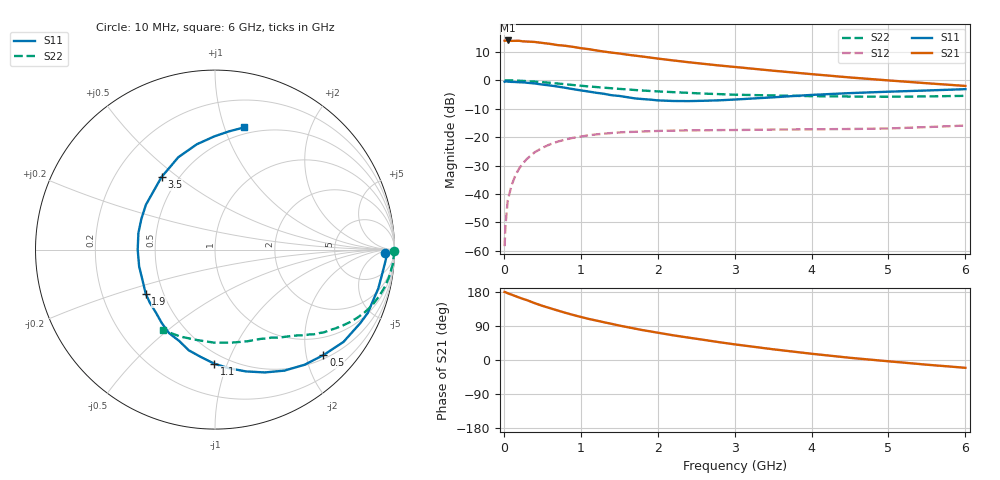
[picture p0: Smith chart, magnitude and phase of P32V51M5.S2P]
! SIEMENS Small Signal Semiconductors
! BFP181
! Si NPN RF Bipolar Junction Transistor in SOT143
! VCE = 2.5 V  IC = 1.5 mA
! Common Emitter S-Parameters:  March  1996
# GHz  S  MA  R  50
!  f  S11  S21  S12  S22
! GHz  MAG  ANG  MAG  ANG  MAG  ANG  MAG  ANG
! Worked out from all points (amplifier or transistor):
!   36 points, 10 MHz to 6 GHz, reference 50 ohm
!   highest |S21| = 14.1 dB at 50 MHz (marker M1)
!   |S21| within 3 dB of that: start of sweep to 1.086 GHz
!   unconditionally stable (mu >= 1): 2.69 GHz to end of sweep
!   at 250 MHz: K = 0.11, MSG = 21.4 dB, |S12| = -29.2 dB
!   at 1.4 GHz: K = 0.58, MSG = 14.2 dB, |S12| = -18.6 dB
!   at 6 GHz: K = 1.18, MAG = 4.4 dB, |S12| = -15.9 dB
!   S11 on the Smith chart (normalised r, x): 10 MHz: 31, -11; 500 MHz: 0.58, -2.34; 1.1 GHz: 0.42, -0.90; 1.9 GHz: 0.40, -0.25; 3.5 GHz: 0.40, +0.44; 6 GHz: 0.44, +1.17
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0.01  0.9447 -1.2  4.986 179.5  0.0012 90.4  0.9978 -0.3
0.02  0.9578 -1.9  5.023 179.0  0.0026 81.4  0.9975 -0.9
0.05  0.9502 -4.4  5.041 176.2  0.0076 89.5  0.9961 -2.0
0.1  0.9394 -9.4  4.957 172.5  0.0141 81.9  0.9955 -4.1
0.2  0.9248 -18.2  4.973 164.8  0.0281 78.6  0.9846 -8.2
0.4  0.8814 -35.7  4.743 150.0  0.054 67.7  0.9507 -15.9
0.5  0.8429 -44.2  4.56 143.0  0.0647 62.3  0.929 -19.5
0.6  0.8129 -52.1  4.389 136.8  0.0747 58.0  0.9046 -22.7
0.8  0.7386 -67.9  4.059 124.6  0.0908 49.8  0.8542 -28.2
0.9  0.7 -75.8  3.886 118.9  0.0972 45.9  0.8278 -30.7
1.1  0.6353 -90.4  3.549 108.6  0.1078 39.7  0.7812 -35.1
1.3  0.5799 -104.6  3.215 99.7  0.115 34.0  0.7429 -38.8
1.5  0.5314 -118.7  2.971 90.9  0.1208 29.8  0.7068 -42.0
1.8  0.4684 -140.8  2.628 79.0  0.1258 24.6  0.6624 -46.2
1.9  0.4582 -147.3  2.524 75.6  0.1267 22.8  0.6496 -47.7
2.2  0.4329 -167.6  2.244 65.2  0.1302 19.0  0.6196 -51.8
2.8  0.4445 157.4  1.826 47.0  0.133 13.8  0.5721 -60.0
3.5  0.5022 126.4  1.479 28.3  0.1358 10.1  0.5415 -70.7
4  0.554 111.6  1.286 16.5  0.1372 8.2  0.5264 -80.0
4.5  0.5958 99.7  1.124 5.8  0.139 7.1  0.5188 -90.2
5.5  0.6626 83.4  0.889 -12.4  0.1503 7.5  0.5215 -111.6
6  0.6991 76.7  0.797 -20.6  0.1599 6.6  0.5334 -122.6
